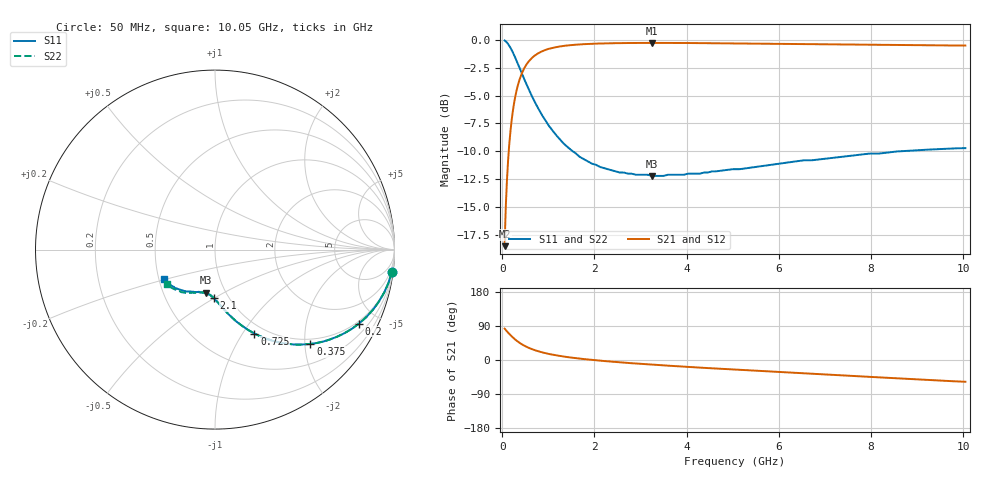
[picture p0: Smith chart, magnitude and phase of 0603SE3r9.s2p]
! AVX Thin Film Operation		Date: August 2001
! Description: Accu-P® Series, Thin Film, SMD, RF Capacitor
! Part Number: 06035J3R9ABT
! 50 MHz  -  10.05 GHz
! Serial Measurements
# mhz S db R 50
!	S11		S21		S12		S22
!	dB	Phase	dB	Phase	dB	Phase	dB	Phase
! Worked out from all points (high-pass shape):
!   401 points, 50 MHz to 10.05 GHz, reference 50 ohm
!   highest |S21| = -0.28 dB at 3.25 GHz (marker M1); lowest = -18.5 dB at 50 MHz (marker M2)
!   |S21| within 3 dB of the highest: 398.7 MHz to end of sweep
!   lowest |S11| = -12.2 dB at 3.25 GHz (marker M3), VSWR 1.65, Z = 40.4 - j20.6 ohm
!   |S11| at or under -10 dB: 1.531 GHz to 8.594 GHz (7.064 GHz wide, 140 % of centre)
!   |S22| runs from -12.1 to -0.1 dB; largest |S21 - S12| = 0
!   S11 on the Smith chart (normalised r, x): 50 MHz: 1, -16; 200 MHz: 0.89, -3.95; 375 MHz: 0.89, -2.12; 725 MHz: 0.89, -1.13; 2.1 GHz: 0.85, -0.50; 10.05 GHz: 0.53, -0.20
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50  -0.06 -7.2  -18.50 82.8  -18.50 82.8  -0.06 -7.2
100  -0.24 -14.3  -12.66 75.7  -12.66 75.7  -0.24 -14.3
125  -0.38 -17.7  -10.86 72.3  -10.86 72.3  -0.38 -17.7
150  -0.53 -21.0  -9.41 69.0  -9.41 69.0  -0.53 -21.0
200  -0.89 -27.1  -7.31 62.9  -7.31 62.9  -0.89 -27.1
275  -1.55 -35.4  -5.23 54.5  -5.23 54.5  -1.55 -35.4
375  -2.52 -44.7  -3.56 45.3  -3.56 45.3  -2.52 -44.7
525  -3.99 -55.1  -2.21 34.8  -2.21 34.8  -3.99 -55.1
625  -4.90 -60.4  -1.70 29.5  -1.70 29.5  -4.90 -60.4
725  -5.73 -64.8  -1.36 25.2  -1.36 25.2  -5.73 -64.8
900  -7.00 -70.9  -0.97 19.1  -0.97 19.1  -7.00 -70.8
1125  -8.32 -76.6  -0.70 13.4  -0.70 13.4  -8.32 -76.5
1375  -9.46 -81.7  -0.53 8.3  -0.53 8.3  -9.46 -81.5
1725  -10.60 -87.0  -0.40 3.1  -0.40 3.1  -10.60 -86.7
2100  -11.36 -91.5  -0.34 -1.5  -0.34 -1.5  -11.36 -91.1
2550  -11.90 -96.2  -0.30 -6.1  -0.30 -6.1  -11.90 -95.6
3250  -12.20 -102.1  -0.28 -12.3  -0.28 -12.3  -12.10 -101.1
3400  -12.20 -103.8  -0.28 -13.4  -0.28 -13.4  -12.10 -102.8
5050  -11.60 -116.4  -0.33 -25.5  -0.33 -25.5  -11.56 -114.4
6725  -10.80 -128.0  -0.40 -36.5  -0.40 -36.5  -10.70 -124.0
8400  -10.09 -139.2  -0.47 -47.2  -0.47 -47.2  -10.09 -134.2
10050  -9.71 -149.8  -0.52 -57.5  -0.52 -57.5  -9.68 -143.8
